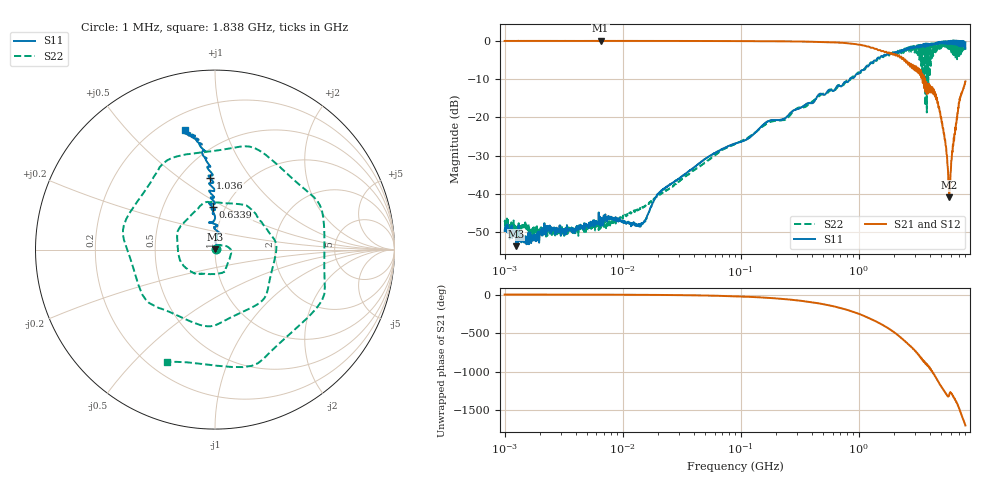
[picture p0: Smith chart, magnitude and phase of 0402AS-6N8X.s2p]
!s-Parameter Generated by FASTRON Sdn. Bhd.
!FASTRON P/N : 0402AS-6N8X
!Keysight Technologies: E5071C_MY46733604_B.14.02
!Date: Mon Dec 01 10:25:24 2025
!Version  :Rev00  Mon Dec 01 10:25:24 2025
!Data & Calibration Information:
!Freq  S11:SOLT2(ON)  S21:SOLT2(ON)  S12:SOLT2(ON)  S22:SOLT2(ON)
!PortZ  Port1:50+j0  Port2:50+j0
!When reading reference impedance value at option line is always used.
! Remarks : This data is being provided solely for informational purposes.
# Hz S dB R 50
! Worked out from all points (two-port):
!   1601 points, 1 MHz to 8 GHz, reference 50 ohm
!   highest |S21| = 0.01 dB at 6.499 MHz (marker M1); lowest = -40.8 dB at 5.841 GHz (marker M2)
!   |S21| within 3 dB of the highest: start of sweep to 1.724 GHz
!   lowest |S11| = -53.6 dB at 1.251 MHz (marker M3), VSWR 1.00, Z = 50.2 + j0.0853 ohm
!   |S11| at or under -10 dB: start of sweep to 840.5 MHz
!   |S22| runs from -51.1 to -0.6 dB; largest |S21 - S12| = 0.021
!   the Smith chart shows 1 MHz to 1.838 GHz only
!   S11 on the Smith chart (normalised r, x): 1 MHz: 1.01, +0.00; 633.9 MHz: 0.87, +0.44; 1.036 GHz: 0.69, +0.66; 1.838 GHz: 0.29, +0.74
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1000000  -49.60 14.3  -0.04 -0.3  -0.02 -0.3  -47.30 21.5
1250831  -53.60 24.0  -0.05 -0.3  -0.03 -0.3  -49.50 9.9
4479405  -48.20 33.4  -0.04 -1.2  -0.02 -1.2  -49.30 40.2
6498814  -48.40 51.0  0.01 -2.0  -0.06 -1.5  -47.10 43.6
2.00676e7  -39.80 49.9  -0.04 -5.2  -0.04 -5.1  -40.30 68.8
8.994653e7  -26.80 89.0  -0.08 -22.8  -0.07 -22.8  -26.90 30.1
4.006501e8  -16.30 98.3  -0.25 -100.0  -0.24 -100.0  -15.90 -122.0
6.339096e8  -12.50 92.9  -0.43 -158.0  -0.43 -158.0  -12.80 130.0
1.035959e9  -7.99 93.9  -1.05 101.0  -1.05 101.0  -8.34 -73.0
1.442356e9  -4.50 98.5  -2.34 0.5  -2.33 0.4  -4.77 79.4
1.7949e9  -3.65 103.0  -3.03 -82.0  -3.04 -82.1  -3.78 -89.0
1.83751e9  -3.28 104.0  -3.32 -93.2  -3.32 -93.3  -3.36 -113.0
2.157084e9  -2.93 108.0  -4.04 -169.0  -4.03 -169.0  -2.67 94.6
2.516241e9  -1.99 115.0  -5.66 101.0  -5.63 100.0  -2.23 -98.1
2.868376e9  -1.91 121.0  -6.24 20.6  -6.21 20.5  -2.74 99.6
3.244011e9  -1.72 128.0  -7.28 -67.9  -7.25 -68.1  -2.23 -76.2
3.60885e9  -1.28 137.0  -10.90 -147.0  -10.90 -148.0  -1.56 85.8
4.034495e9  -0.98 143.0  -12.80 110.0  -12.80 109.0  -1.57 -93.4
4.352635e9  -0.70 146.0  -14.10 42.1  -14.10 41.5  -2.94 119.0
4.716529e9  -0.70 153.0  -17.00 -51.9  -17.00 -52.4  -1.09 -82.5
5.840928e9  -0.08 -165.0  -40.80 145.0  -40.90 145.0  -1.53 98.4
8e9  -0.41 -100.0  -10.60 103.0  -10.70 103.0  -2.37 141.0
